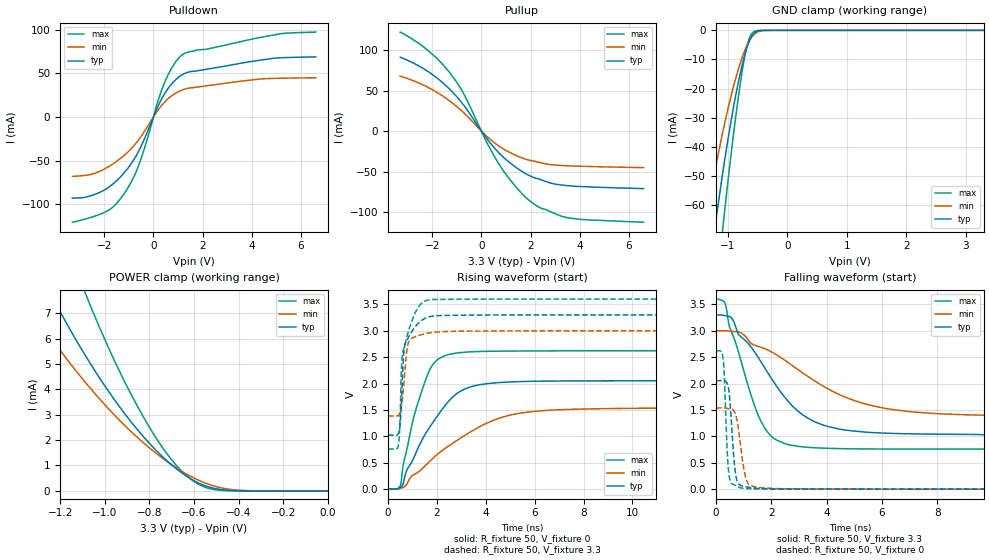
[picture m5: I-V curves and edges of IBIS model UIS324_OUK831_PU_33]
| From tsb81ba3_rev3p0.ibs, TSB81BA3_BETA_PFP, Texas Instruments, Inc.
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[Model]   UIS324_OUK831_PU_33
Model_type  I/O
Enable   Active-High
Vref =   0
Rref =   500
Cref =   10p
Vmeas =   1.65
| variable   typ   min   max
C_comp   1.99pF   1.39pF   3.76pF
| C_pullup   4.47pF   1.87pF   5.41pF
| C_pulldown   4.72pF   1.53pF   7.50pF
| C_tri-state   1.99pF   1.39pF   3.76pF
[Temperature Range]   40   125   -40
| Ambient temperature   25   110   -40
[Voltage range]   3.3   3   3.6
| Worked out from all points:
|   slope of the pulldown table from 0 to 0.495 V, typ, clamps not added: 17.4 ohm
|   slope of the pullup table from 0 to 0.495 V, typ, clamps not added: 25.3 ohm
|   GND clamp passes 1 mA (typ) near -0.56 V on its own axis
|   POWER clamp passes 1 mA (typ) near -0.70 V on its own axis
|   rising waveform, R_fixture 50, V_fixture 0: 20-80 % time 1.61ns typ, 2.77ns min, 911ps max; typ from 0 V to 2.06 V
|   falling waveform, R_fixture 50, V_fixture 3.3: 20-80 % time 1.97ns typ, 3.17ns min, 1.07ns max; typ from 3.3 V to 1.02 V
|   rising waveform, R_fixture 50, V_fixture 3.3: 20-80 % time 269ps typ, 202ps min, 369ps max; typ from 1.02 V to 3.3 V
|   falling waveform, R_fixture 50, V_fixture 0: 20-80 % time 172ps typ, 251ps min, 122ps max; typ from 2.06 V to 0 V
[GND Clamp]
| UIS324_OUK831_PU_33
|   Voltage   I(typ)   I(min)   I(max)
-3.3V     -469.1mA   -362mA     -576.5mA
-1.41V    -98.24mA   -69.95mA   -134.9mA
-1.375V   -92.48mA   -65.8mA    -127.3mA
-1.205V   -65.9mA    -46.84mA   -91.61mA
-1.08V    -48.08mA   -34.35mA   -66.9mA
-895mV    -25.2mA    -18.49mA   -34mA
-750mV    -11.1mA    -8.76mA    -12.82mA
-655mV    -4.534mA   -4.177mA   -3.665mA
-610mV    -2.448mA   -2.634mA   -1.492mA
-550mV    -834.8uA   -1.235mA   -325.2uA
-240mV    -10.16uA   -12.08uA   -10uA
3.3V      -10uA      -7.002uA   -10uA
[POWER Clamp]
| UIS324_OUK831_PU_33
|   Voltage   I(typ)   I(min)   I(max)
-3.3V     62.68mA    47.7mA     84.8mA
-1.38V    10.19mA    7.838mA    15.05mA
-1.235V   7.641mA    5.966mA    11.26mA
-1.095V   5.455mA    4.363mA    7.97mA
-1.075V   5.167mA    4.151mA    7.533mA
-940mV    3.389mA    2.836mA    4.826mA
-810mV    1.969mA    1.767mA    2.656mA
-705mV    1.055mA    1.055mA    1.27mA
-615mV    469.2uA    567.9uA    456.5uA
-535mV    147.8uA    252.9uA    93.07uA
-415mV    606.1nA    28.94uA    -7.324uA
-48.03fV  -10uA      -9.994uA   -10uA
[Pulldown]
| UIS324_OUK831_PU_33
|   Voltage   I(typ)   I(min)   I(max)
-3.3V     -92.9mA    -68.01mA   -120.4mA
-2.64V    -90.95mA   -66.29mA   -115.7mA
-1.855V   -81.13mA   -57.35mA   -107.2mA
-1.135V   -61.97mA   -42.51mA   -85.32mA
-570mV    -37.33mA   -24.91mA   -52.89mA
-240mV    -16.7mA    -10.89mA   -24.29mA
180mV     12mA       7.634mA    17.88mA
445mV     26.17mA    16.71mA    38.83mA
790mV     39.4mA     25.18mA    58.31mA
1.15V     48.05mA    30.64mA    70.82mA
5.11V     67.66mA    44.28mA    94.91mA
6.6V      68.79mA    44.92mA    97.14mA
[Pullup]
| UIS324_OUK831_PU_33
|   Voltage   I(typ)   I(min)   I(max)
-3.3V     91.06mA    67.68mA    122.1mA
-2.15V    73.02mA    53.59mA    98.88mA
-1.67V    62.17mA    45.17mA    85.36mA
-1.245V   50.31mA    36.14mA    70.38mA
-680mV    30.42mA    21.53mA    43.84mA
200mV     -8.418mA   -5.847mA   -12.61mA
710mV     -26.75mA   -18.34mA   -40.44mA
1.4V      -44.59mA   -29.91mA   -68.56mA
2V        -55.49mA   -36.31mA   -86.83mA
2.475V    -60.58mA   -39.54mA   -95.81mA
3.465V    -67.12mA   -42.73mA   -106.5mA
6.6V      -70.9mA    -45.03mA   -112.3mA
[Ramp]
| UIS324_OUK831_PU_33
| variable   typ   min   max
dV/dt_r   1.23/1.61E-09   0.92/2.77E-09   1.57/9.12E-10
dV/dt_f   1.37/1.97E-09   0.97/3.18E-09   1.71/1.08E-09
R_load = 50
[Rising Waveform]
| UIS324_OUK831_PU_33
R_fixture =   50
C_fixture =   0
L_fixture =   0
V_fixture =   0
V_fixture_min = 0
V_fixture_max = 0
|   Time   V(typ)   V(min)   V(max)
0s        74.15uV    43.33uV    60.76uV
510ps     33.13mV    16.61mV    79.53mV
635ps     134.4mV    36.63mV    492.9mV
1.05ns    593.1mV    272.7mV    1.358V
1.71ns    1.177V     528.7mV    2.266V
2.11ns    1.446V     694.1mV    2.479V
2.815ns   1.81V      922mV      2.578V
4.72ns    2.024V     1.369V     2.615V
7.07ns    2.049V     1.506V     2.619V
40ns      2.055V     1.538V     2.624V
[Falling Waveform]
| UIS324_OUK831_PU_33
R_fixture =   50
C_fixture =   0
L_fixture =   0
V_fixture =   3.3
V_fixture_min = 3
V_fixture_max = 3.6
|   Time   V(typ)   V(min)   V(max)
0s        3.3V       3V         3.6V
330ps     3.285V     3V         3.512V
495ps     3.268V     2.992V     3.063V
1.695ns   2.354V     2.675V     1.218V
2.13ns    1.997V     2.563V     948.4mV
2.935ns   1.491V     2.276V     813.4mV
3.885ns   1.212V     1.948V     776.4mV
5.225ns   1.089V     1.64V      762.7mV
8.2ns     1.04V      1.425V     758.9mV
40ns      1.023V     1.385V     758.3mV
[Rising Waveform]
| UIS324_OUK831_PU_33
R_fixture =   50
C_fixture =   0
L_fixture =   0
V_fixture =   3.3
V_fixture_min = 3
V_fixture_max = 3.6
|   Time   V(typ)   V(min)   V(max)
0s        1.023V     1.385V     758.3mV
425ps     1.058V     1.401V     835.4mV
480ps     1.176V     1.444V     1.187V
555ps     1.723V     1.603V     2.359V
625ps     2.447V     1.887V     2.639V
755ps     2.81V      2.566V     2.858V
860ps     2.896V     2.802V     3.033V
1.23ns    3.138V     2.905V     3.44V
1.635ns   3.258V     2.955V     3.581V
40ns      3.3V       3V         3.6V
[Falling Waveform]
| UIS324_OUK831_PU_33
R_fixture =   50
C_fixture =   0
L_fixture =   0
V_fixture =   0
V_fixture_min = 0
V_fixture_max = 0
|   Time   V(typ)   V(min)   V(max)
0s        2.055V     1.538V     2.624V
190ps     2.052V     1.538V     2.609V
270ps     2.049V     1.538V     2.414V
415ps     1.989V     1.527V     627.8mV
490ps     1.751V     1.52V      207.8mV
705ps     304.5mV    1.421V     71.12mV
955ps     58.57mV    559.9mV    18.78mV
1.21ns    31.98mV    75.36mV    9.322mV
2.215ns   5.241mV    10.91mV    2.202mV
40ns      89.02uV    121.6uV    63.13uV
